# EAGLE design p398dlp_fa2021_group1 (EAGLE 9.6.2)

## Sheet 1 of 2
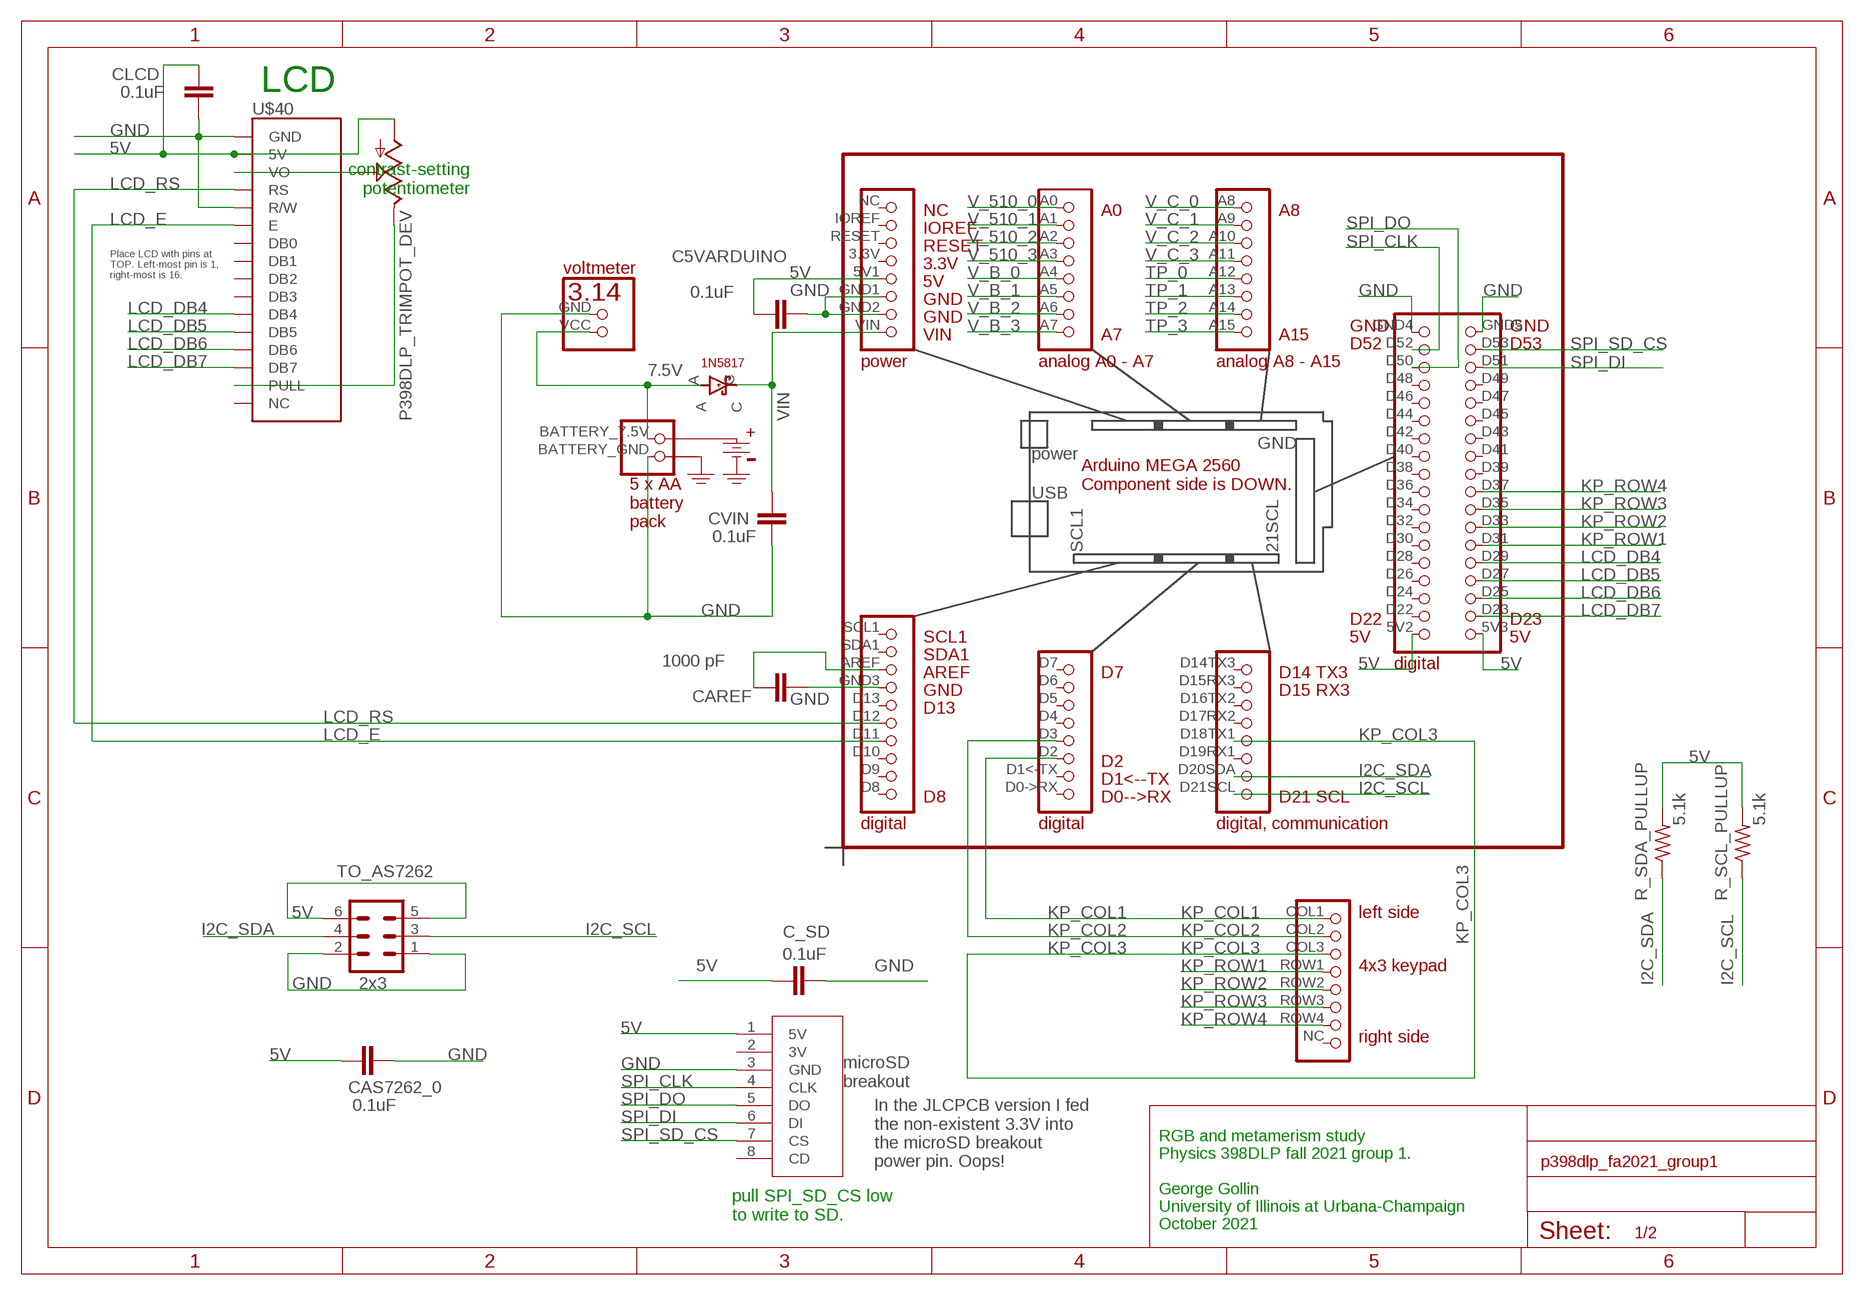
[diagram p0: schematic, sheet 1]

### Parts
C5VARDUINO  0.1uF  C5/3.5  [C5B3.5]
C_SD  0.1uF  C5/3.5  [C5B3.5]
CAREF  1000 pF  C5/3.5  [C5B3.5]
CAS7262_0  0.1uF  C5/3.5  [C5B3.5]
CLCD  0.1uF  C5/3.5  [C5B3.5]
CVIN  0.1uF  C5/3.5  [C5B3.5]
DIODE1  P398DLP_1N5817_DEV  [P398DLP_1N5817_PKG]
R_SCL_PULLUP  5.1k  R-US_0207/7  [0207/7]
R_SDA_PULLUP  5.1k  R-US_0207/7  [0207/7]
TO_AS7262  2x3  P398DLP_RIBBON_PCB_2X3_DEV  [06V]
U$1  P398DLP_5XAA_BATTERY_DEV  [P398DLP_5XAA_BATTERY_PKG]
U$2  P398DLP_KEYPAD_DEV  [P398DLP_KEYPAD_PKG]
U$3  P398DLP_VOLTMETER_DEV  [P398DLP_VOLTMETER_PKG]
U$5  P398DLP_ARDUINO_MEGA2560_DEV  [P398DLP_ARDUINO_MEGA2560_PKG]
U$19  P398DLP_TRIMPOT_DEV  [P398DLP_TRIMPOT_PKG]
U$40  P398DLP_LCD_16X2_DEV  [P398DLP_LCD_16X2_PKG]
U$MICROSD  P398DLP_MICROSD_DEV  [P398DLP_MICROSD_PKG]

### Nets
5V [power]: C5VARDUINO.1 C_SD.2 CAS7262_0.1 CLCD.1 R_SCL_PULLUP.2 R_SDA_PULLUP.2 TO_AS7262.5 TO_AS7262.6 U$5.5V1 U$5.5V2 U$5.5V3 U$19.BOTTOM U$40.5V U$MICROSD.1(5V) ; also sheet 2
7.5V [power]: DIODE1.A U$1.BATTERY_7.5V U$3.VCC
AREF: CAREF.1 U$5.AREF
GND [power]: C5VARDUINO.2 C_SD.1 CAREF.2 CAS7262_0.2 CLCD.2 CVIN.1 TO_AS7262.1 TO_AS7262.2 U$1.BATTERY_GND U$3.GND U$5.GND1 U$5.GND2 U$5.GND3 U$5.GND4 U$5.GND5 U$40.GND U$40.R/W U$MICROSD.3(GND) ; also sheet 2
I2C_SCL: R_SCL_PULLUP.1 TO_AS7262.3 U$5.D21SCL ; also sheet 2
I2C_SDA: R_SDA_PULLUP.1 TO_AS7262.4 U$5.D20SDA ; also sheet 2
KP_COL1: U$2.COL1 U$5.D2
KP_COL2: U$2.COL2 U$5.D3
KP_COL3: U$2.COL3 U$5.D18TX1
KP_ROW1: U$2.ROW1 U$5.D31
KP_ROW2: U$2.ROW2 U$5.D33
KP_ROW3: U$2.ROW3 U$5.D35
KP_ROW4: U$2.ROW4 U$5.D37
LCD_DB4: U$5.D29 U$40.DB4
LCD_DB5: U$5.D27 U$40.DB5
LCD_DB6: U$5.D25 U$40.DB6
LCD_DB7: U$5.D23 U$40.DB7
LCD_E: U$5.D11 U$40.E
LCD_RS: U$5.D12 U$40.RS
LCD_VEE: U$19.TOP U$40.PULL
N$6: U$19.TAP U$40.VO
SPI_CLK: U$5.D52 U$MICROSD.4(CLK)
SPI_DI: U$5.D51 U$MICROSD.6(DI)
SPI_DO: U$5.D50 U$MICROSD.5(DO)
SPI_SD_CS: U$5.D53 U$MICROSD.7(CS)
TP_0: U$5.A12 ; also sheet 2
TP_1: U$5.A13 ; also sheet 2
TP_2: U$5.A14 ; also sheet 2
TP_3: U$5.A15 ; also sheet 2
V_510_0: U$5.A0 ; also sheet 2
V_510_1: U$5.A1 ; also sheet 2
V_510_2: U$5.A2 ; also sheet 2
V_510_3: U$5.A3 ; also sheet 2
V_B_0: U$5.A4 ; also sheet 2
V_B_1: U$5.A5 ; also sheet 2
V_B_2: U$5.A6 ; also sheet 2
V_B_3: U$5.A7 ; also sheet 2
V_C_0: U$5.A8 ; also sheet 2
V_C_1: U$5.A9 ; also sheet 2
V_C_2: U$5.A10 ; also sheet 2
V_C_3: U$5.A11 ; also sheet 2
VIN: CVIN.2 DIODE1.C U$5.VIN
Unconnected: U$2.NC U$5.3.3V U$5.D0->RX U$5.D1<-TX U$5.D4 U$5.D5 U$5.D6 U$5.D7 U$5.D8 U$5.D9 U$5.D10 U$5.D13 U$5.D14TX3 U$5.D15RX3 U$5.D16TX2 U$5.D17RX2 U$5.D19RX1 U$5.D22 U$5.D24 U$5.D26 U$5.D28 U$5.D30 U$5.D32 U$5.D34 U$5.D36 U$5.D38 U$5.D39 U$5.D40 U$5.D41 U$5.D42 U$5.D43 U$5.D44 U$5.D45 U$5.D46 U$5.D47 U$5.D48 U$5.D49 U$5.IOREF U$5.NC U$5.RESET U$5.SCL1 U$5.SDA1 U$40.DB0 U$40.DB1 U$40.DB2 U$40.DB3 U$40.NC U$MICROSD.2(3V) U$MICROSD.8(CD)

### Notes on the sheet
- LCD
- contrast-setting
  potentiometer
- Place LCD with pins at 
  TOP. Left-most pin is 1, 
  right-most is 16.
- In the JLCPCB version I fed 
  the non-existent 3.3V into 
  the microSD breakout 
  power pin. Oops!
- pull SPI_SD_CS low
  to write to SD.
- RGB and metamerism study
  Physics 398DLP fall 2021 group 1.
  
  George Gollin
  University of Illinois at Urbana-Champaign
  October 2021

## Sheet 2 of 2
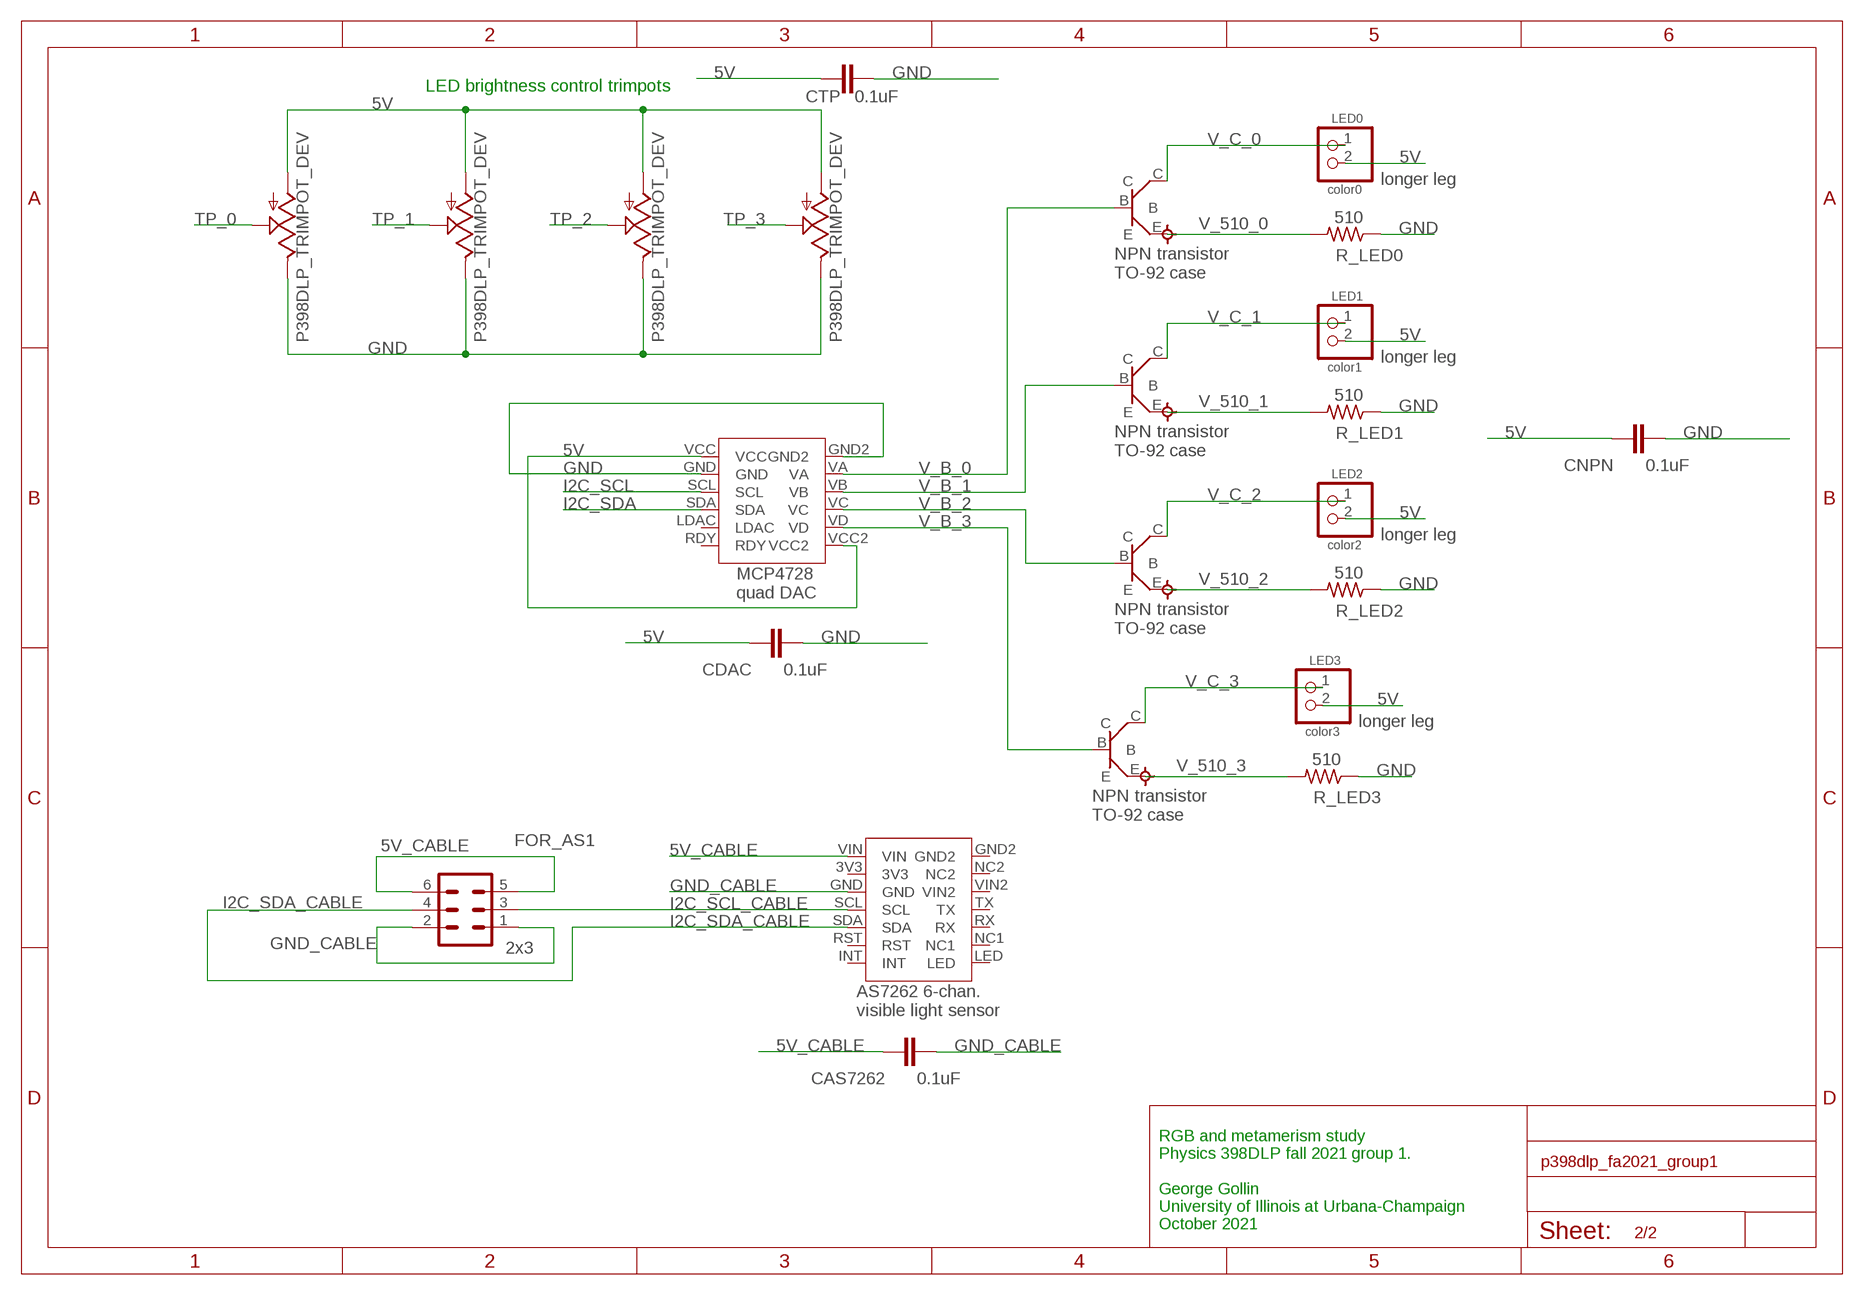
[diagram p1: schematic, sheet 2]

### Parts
CAS7262  0.1uF  C5/3.5  [C5B3.5]
CDAC  0.1uF  C5/3.5  [C5B3.5]
CNPN  0.1uF  C5/3.5  [C5B3.5]
CTP  0.1uF  C5/3.5  [C5B3.5]
FOR_AS1  2x3  P398DLP_RIBBON_PCB_2X3_DEV  [06V]
LED0  color0  PINHD-1X2  [1X02]
LED1  color1  PINHD-1X2  [1X02]
LED2  color2  PINHD-1X2  [1X02]
LED3  color3  PINHD-1X2  [1X02]
NPN0  P398DLP_NPN_DEV  [P398DLP_NPN_PKG]
NPN1  P398DLP_NPN_DEV  [P398DLP_NPN_PKG]
NPN2  P398DLP_NPN_DEV  [P398DLP_NPN_PKG]
NPN3  P398DLP_NPN_DEV  [P398DLP_NPN_PKG]
R_LED0  510  R-US_0207/7  [0207/7]
R_LED1  510  R-US_0207/7  [0207/7]
R_LED2  510  R-US_0207/7  [0207/7]
R_LED3  510  R-US_0207/7  [0207/7]
U$4  P398DLP_AS7262_DEV  [P398DLP_AS7262_PKG]
U$6  P398DLP_MCP4728_DEV  [P398DLP_MCP4728_PKG]
U$8  P398DLP_TRIMPOT_DEV  [P398DLP_TRIMPOT_PKG]
U$12  P398DLP_TRIMPOT_DEV  [P398DLP_TRIMPOT_PKG]
U$13  P398DLP_TRIMPOT_DEV  [P398DLP_TRIMPOT_PKG]
U$14  P398DLP_TRIMPOT_DEV  [P398DLP_TRIMPOT_PKG]

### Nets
5V [power]: CDAC.2 CNPN.2 CTP.2 LED0.2 LED1.2 LED2.2 LED3.2 U$6.VCC U$6.VCC2 U$8.BOTTOM U$12.BOTTOM U$13.BOTTOM U$14.BOTTOM ; also sheet 1
5V_CABLE: CAS7262.2 FOR_AS1.5 FOR_AS1.6 U$4.VIN
GND [power]: CDAC.1 CNPN.1 CTP.1 R_LED0.1 R_LED1.1 R_LED2.1 R_LED3.1 U$6.GND U$6.GND2 U$8.TOP U$12.TOP U$13.TOP U$14.TOP ; also sheet 1
GND_CABLE: CAS7262.1 FOR_AS1.1 FOR_AS1.2 U$4.GND
I2C_SCL: U$6.SCL ; also sheet 1
I2C_SCL_CABLE: FOR_AS1.3 U$4.SCL
I2C_SDA: U$6.SDA ; also sheet 1
I2C_SDA_CABLE: FOR_AS1.4 U$4.SDA
TP_0: U$8.TAP ; also sheet 1
TP_1: U$12.TAP ; also sheet 1
TP_2: U$13.TAP ; also sheet 1
TP_3: U$14.TAP ; also sheet 1
V_510_0: NPN0.E R_LED0.2 ; also sheet 1
V_510_1: NPN1.E R_LED1.2 ; also sheet 1
V_510_2: NPN2.E R_LED2.2 ; also sheet 1
V_510_3: NPN3.E R_LED3.2 ; also sheet 1
V_B_0: NPN0.B U$6.VA ; also sheet 1
V_B_1: NPN1.B U$6.VB ; also sheet 1
V_B_2: NPN2.B U$6.VC ; also sheet 1
V_B_3: NPN3.B U$6.VD ; also sheet 1
V_C_0: LED0.1 NPN0.C ; also sheet 1
V_C_1: LED1.1 NPN1.C ; also sheet 1
V_C_2: LED2.1 NPN2.C ; also sheet 1
V_C_3: LED3.1 NPN3.C ; also sheet 1
Unconnected: U$4.3V3 U$4.GND2 U$4.INT U$4.LED U$4.NC1 U$4.NC2 U$4.RST U$4.RX U$4.TX U$4.VIN2 U$6.LDAC U$6.RDY

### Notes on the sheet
- LED brightness control trimpots
- longer leg
- longer leg
- longer leg
- longer leg
- RGB and metamerism study
  Physics 398DLP fall 2021 group 1.
  
  George Gollin
  University of Illinois at Urbana-Champaign
  October 2021

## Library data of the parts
C5VARDUINO C_SD CAREF CAS7262 CAS7262_0 CDAC CLCD CNPN CTP CVIN = capacitor-wima:C: CAPACITOR
DIODE1 = p398dlp:P398DLP_1N5817_DEV: 1N5817 Schottky barrier diode
FOR_AS1 TO_AS7262 = p398dlp:P398DLP_RIBBON_PCB_2X3_DEV: CONNECTOR; OC_FARNELL: unknown; OC_NEWARK: unknown
LED0 LED1-LED3 = p398dlp_sp2020:PINHD-1X2: PIN HEADER
NPN0 NPN1-NPN3 = p398dlp:P398DLP_NPN_DEV: NPN transistor, TO-92 case
R_LED0 R_LED1-R_LED3 R_SCL_PULLUP R_SDA_PULLUP = resistor:R-US_: RESISTOR, American symbol
U$1 = p398dlp:P398DLP_5XAA_BATTERY_DEV: 5 x AA battery case
U$2 = p398dlp:P398DLP_KEYPAD_DEV: 3x4 telephone-style keypad
U$3 = p398dlp:P398DLP_VOLTMETER_DEV: Adafruit 2-wire voltmeter
U$4 = p398dlp:P398DLP_AS7262_DEV: AS7262 6 channel visible light sensor
U$5 = p398dlp:P398DLP_ARDUINO_MEGA2560_DEV: Arduino MEGA 2560, component side DOWN
U$6 = p398dlp:P398DLP_MCP4728_DEV: MCP4725 12-bit DACMCP4728 quad 12-bit DAC Adafriuit 4470
U$8 U$12-U$14 U$19 = p398dlp_fa2020:P398DLP_TRIMPOT_DEV: trimpot
U$40 = p398dlp:P398DLP_LCD_16X2_DEV: 2x16 liquid crystal display, four mounting holes
U$MICROSD = p398dlp_sp2020:P398DLP_MICROSD_DEV: Adafruit microSD reader breakout board

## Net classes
1 power: width 0.305 mm

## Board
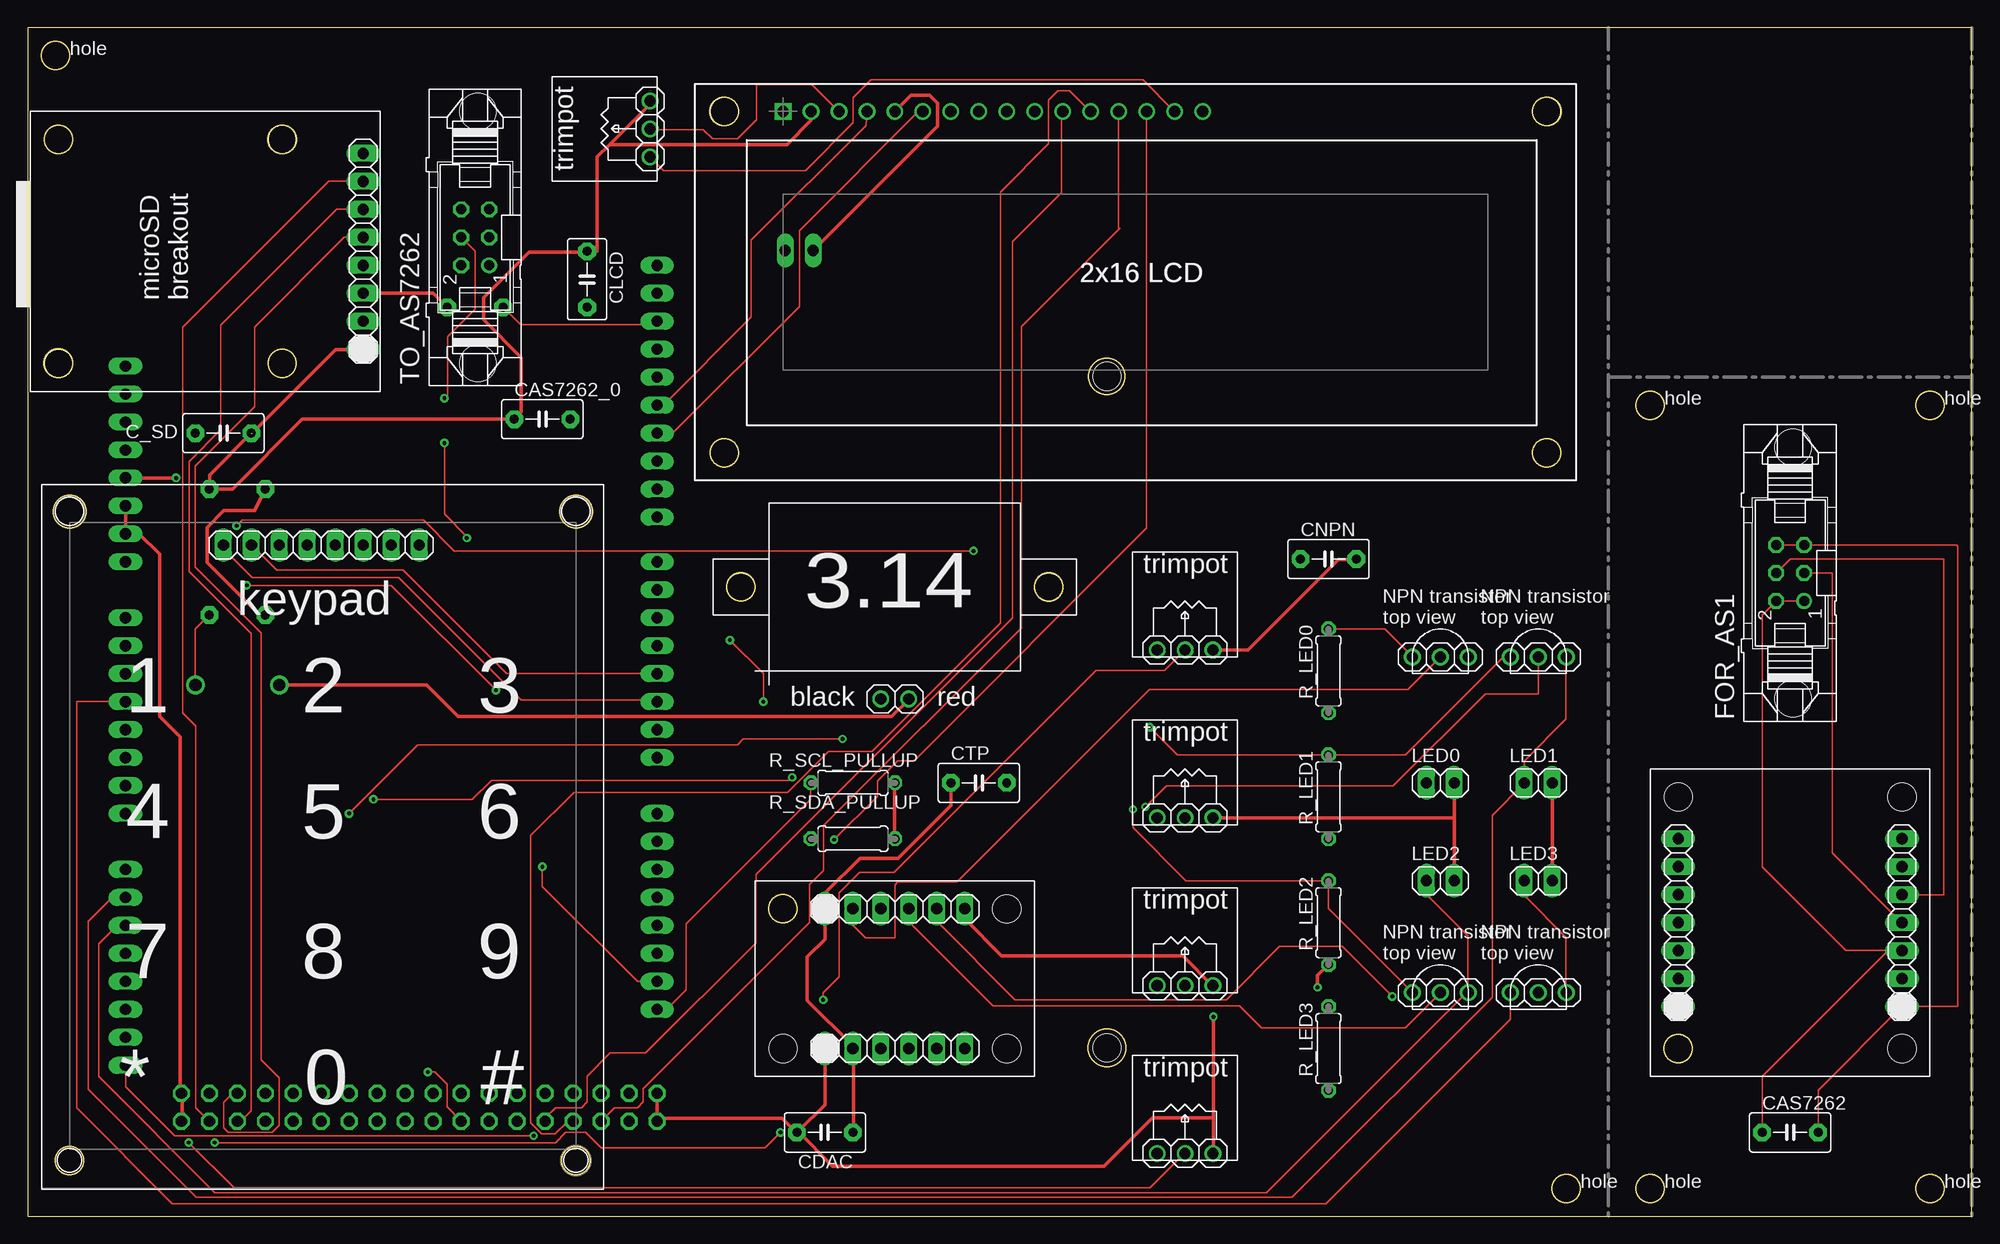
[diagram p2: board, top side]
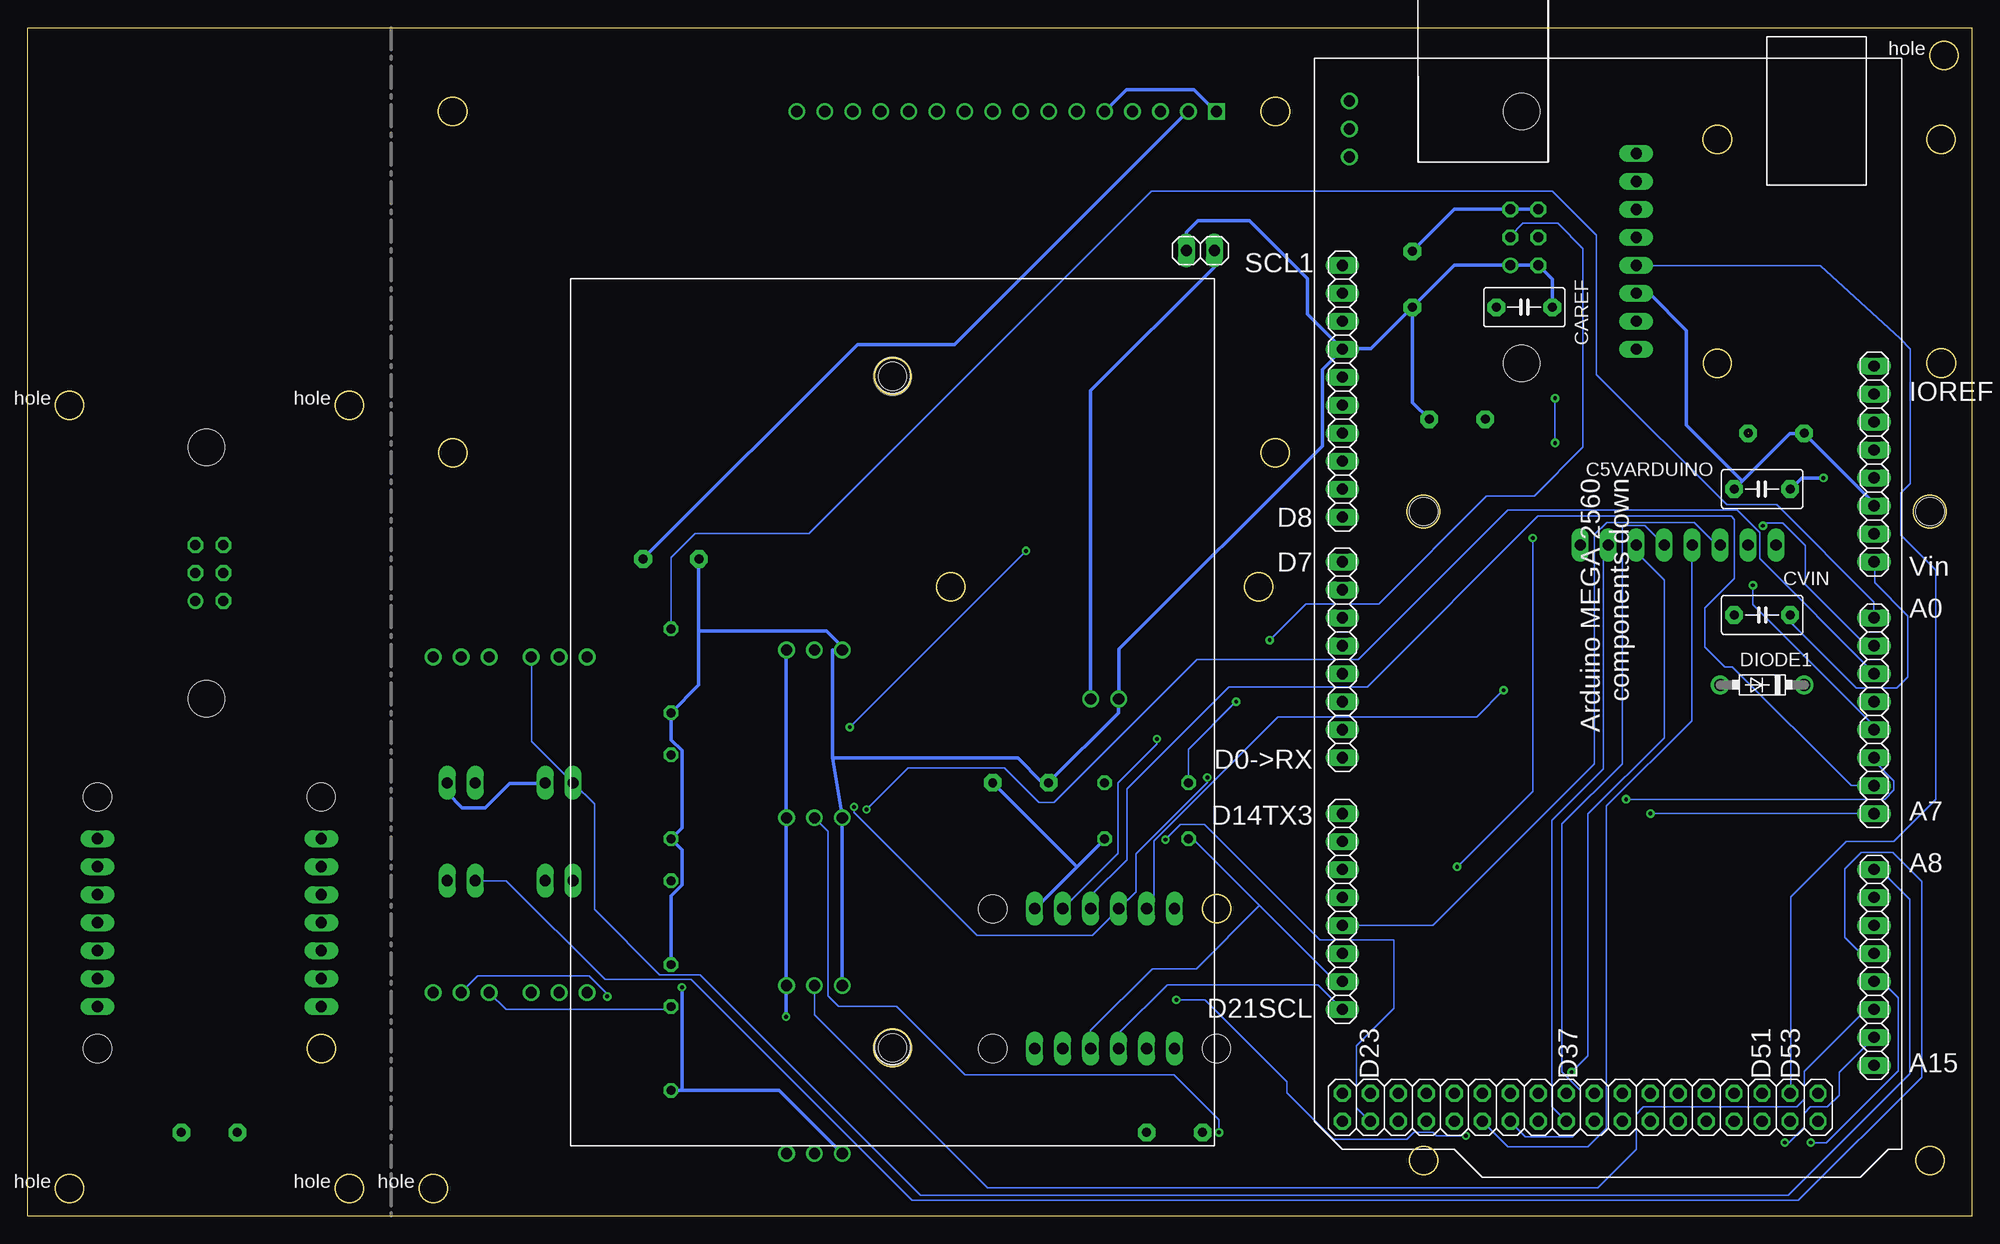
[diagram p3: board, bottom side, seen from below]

Size 176.53 x 107.95 mm. Coordinates in mm from the lower left corner, seen from the top.
Outline: 0,0 176.53,0 176.53,107.95 0,107.95 0,0
Copper layers (1*16): Top 0.035mm / dielectric 1.5mm / Bottom 0.035mm
Design rules "default": minimum track width 6mil, minimum drill 0.35mm, track to track 6mil, track to pad 6mil, pad to pad 6mil, via to via 6mil, smd to smd 6mil, copper to edge 40mil, drill to drill 6mil, minimum pad ring 10mil, minimum via ring 8mil, stop-mask expansion 4mil, vias tented up to drill 0mil, thermal gap 10mil

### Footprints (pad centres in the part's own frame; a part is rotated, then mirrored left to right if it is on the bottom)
C5B3.5 = drill 0.813 pad 1.6 octagon: 1 -2.54,0; 2 2.54,0
P398DLP_1N5817_PKG = drill 1.1 pad 1.7: A -3.81,0; C 3.81,0
06V = drill 0.914: 1 -2.54,-1.27 | drill 0.914 octagon: 2 -2.54,1.27; 3 0,-1.27; 4 0,1.27; 5 2.54,-1.27; 6 2.54,1.27 | hole 3.302: 11.43,-0.254; -11.43,-0.254
1X02 = drill 1.016 long: 1 -1.27,0; 2 1.27,0
P398DLP_NPN_PKG = drill 1.016: B 0,0; C 2.54,0; E -2.54,0
0207/7 = drill 0.813 octagon: 1 -3.81,0; 2 3.81,0
P398DLP_5XAA_BATTERY_PKG = drill 1.016 long: BATTERY_7.5V 0,-2.54; BATTERY_GND 2.54,-2.54 | hole 2.54: 29.21,69.85; 29.21,8.89
P398DLP_KEYPAD_PKG = drill 1.016 long: COL1 0,0; COL2 2.54,0; COL3 5.08,0; NC 17.78,0; ROW1 7.62,0; ROW2 10.16,0; ROW3 12.7,0; ROW4 15.24,0 | hole 2.54: -13.97,3.048; 32.004,3.048; 32.004,-55.88; -13.97,-55.88
P398DLP_VOLTMETER_PKG = drill 1.016: GND 10.16,-2.54; VCC 12.7,-2.54 | hole 2.54: -2.54,7.62; 25.4,7.62
P398DLP_AS7262_PKG = drill 1.016 long: 3V3 8.89,2.54; GND 11.43,2.54; GND2 6.35,22.86; INT 21.59,2.54; LED 21.59,22.86; NC1 19.05,22.86; NC2 8.89,22.86; RST 19.05,2.54; RX 16.51,22.86; SCL 13.97,2.54; SDA 16.51,2.54; TX 13.97,22.86; VIN 6.35,2.54; VIN2 11.43,22.86 | hole 2.54: 2.54,22.86; 25.4,2.54; 25.4,22.86; 2.54,2.54
P398DLP_ARDUINO_MEGA2560_PKG = drill 1.016 long: 3.3V 35.56,50.8; 5V1 38.1,50.8; A0 50.8,50.8; A1 53.34,50.8; A2 55.88,50.8; A3 58.42,50.8; A4 60.96,50.8; A5 63.5,50.8; A6 66.04,50.8; A7 68.58,50.8; A8 73.66,50.8; A9 76.2,50.8; A10 78.74,50.8; A11 81.28,50.8; A12 83.82,50.8; A13 86.36,50.8; A14 88.9,50.8; A15 91.44,50.8; AREF 23.876,2.54; D0->RX 63.5,2.54; D1<-TX 60.96,2.54; D2 58.42,2.54; D3 55.88,2.54; D4 53.34,2.54; D5 50.8,2.54; D6 48.26,2.54; D7 45.72,2.54; D8 41.656,2.54; D9 39.116,2.54; D10 36.576,2.54; D11 34.036,2.54; D12 31.496,2.54; D13 28.956,2.54; D14TX3 68.58,2.54; D15RX3 71.12,2.54; D16TX2 73.66,2.54; D17RX2 76.2,2.54; D18TX1 78.74,2.54; D19RX1 81.28,2.54; D20SDA 83.82,2.54; D21SCL 86.36,2.54; GND1 40.64,50.8; GND2 43.18,50.8; GND3 26.416,2.54; IOREF 30.48,50.8; NC 27.94,50.8; RESET 33.02,50.8; SCL1 18.796,2.54; SDA1 21.336,2.54; VIN 45.72,50.8 | drill 1.016 octagon: 5V2 93.98,2.54; 5V3 96.52,2.54; D22 93.98,5.08; D23 96.52,5.08; D24 93.98,7.62; D25 96.52,7.62; D26 93.98,10.16; D27 96.52,10.16; D28 93.98,12.7; D29 96.52,12.7; D30 93.98,15.24; D31 96.52,15.24; D32 93.98,17.78; D33 96.52,17.78; D34 93.98,20.32; D35 96.52,20.32; D36 93.98,22.86; D37 96.52,22.86; D38 93.98,25.4; D39 96.52,25.4; D40 93.98,27.94; D41 96.52,27.94; D42 93.98,30.48; D43 96.52,30.48; D44 93.98,33.02; D45 96.52,33.02; D46 93.98,35.56; D47 96.52,35.56; D48 93.98,38.1; D49 96.52,38.1; D50 93.98,40.64; D51 96.52,40.64; D52 93.98,43.18; D53 96.52,43.18; GND4 93.98,45.72; GND5 96.52,45.72
P398DLP_MCP4728_PKG = drill 1.016 long: GND 8.89,2.54; GND2 6.35,15.24; LDAC 16.51,2.54; RDY 19.05,2.54; SCL 11.43,2.54; SDA 13.97,2.54; VA 8.89,15.24; VB 11.43,15.24; VC 13.97,15.24; VCC 6.35,2.54; VCC2 19.05,15.24; VD 16.51,15.24 | hole 2.54: 2.54,15.24; 22.86,2.54; 22.86,15.24; 2.54,2.54
P398DLP_MOUNTING_HOLE_PKG = hole 2.54: 0,0
P398DLP_TRIMPOT_PKG = drill 1.016: BOTTOM 7.303,0.635; TAP 4.763,0.635; TOP 2.223,0.635
P398DLP_LCD_16X2_PKG = drill 1.016: 5V 2.544,0.006; DB0 15.244,0.006; DB1 17.784,0.006; DB2 20.324,0.006; DB3 22.864,0.006; DB4 25.404,0.006; DB5 27.944,0.006; DB6 30.484,0.006; DB7 33.024,0.006; E 12.704,0.006; NC 38.104,0.006; PULL 35.564,0.006; R/W 10.164,0.006; RS 7.624,0.006; VO 5.084,0.006 | drill 1.016 square: GND 0.004,0.006 | hole 2.54: -5.334,0; -5.334,-30.988; 69.342,-30.988; 69.342,0
P398DLP_MICROSD_PKG = drill 1.016 long: 1 0,0; 2 2.54,0; 3 5.08,0; 4 7.62,0; 5 10.16,0; 6 12.7,0; 7 15.24,0; 8 17.78,0 | hole 2.54: -1.27,27.686; 19.05,27.686; 19.05,7.366; -1.27,7.366

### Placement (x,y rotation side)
C5VARDUINO  19.05,66.04 180 bottom
C_SD  17.78,71.12 0 top
CAREF  40.64,82.55 0 bottom
CAS7262  160.02,7.62 0 top
CAS7262_0  46.74,72.39 0 top
CDAC  72.39,7.62 180 top
CLCD  50.8,85.09 270 top
CNPN  118.11,59.69 0 top
CTP  86.36,39.37 0 top
CVIN  19.05,54.61 0 bottom
DIODE1  19.05,48.26 0 bottom
FOR_AS1  160.02,58.42 90 top
LED0  128.27,39.37 0 top
LED1  137.16,39.37 0 top
LED2  128.27,30.48 0 top
LED3  137.16,30.48 0 top
NPN0  128.27,50.8 0 top
NPN1  137.16,50.8 0 top
NPN2  128.27,20.32 0 top
NPN3  137.16,20.32 0 top
R_LED0  118.11,49.53 90 top
R_LED1  118.11,38.1 90 top
R_LED2  118.11,26.67 90 top
R_LED3  118.11,15.24 90 top
R_SCL_PULLUP  74.93,39.37 0 top
R_SDA_PULLUP  74.93,34.29 0 top
TO_AS7262  40.64,88.9 90 top
U$1  68.78,85.17 180 bottom
U$2  17.78,60.96 0 top
U$3  67.31,49.53 0 top
U$4  172.72,12.7 90 top
U$5  59.69,105.16 270 bottom
U$6  66.04,12.7 0 top
U$7  [P398DLP_MOUNTING_HOLE_PKG]  172.72,2.54 0 top
U$8  100.33,5.08 0 top
U$9  [P398DLP_MOUNTING_HOLE_PKG]  172.72,73.66 0 top
U$10  [P398DLP_MOUNTING_HOLE_PKG]  147.32,73.66 0 top
U$11  [P398DLP_MOUNTING_HOLE_PKG]  147.32,2.54 0 top
U$12  100.33,20.32 0 top
U$13  100.33,35.56 0 top
U$14  100.33,50.8 0 top
U$19  57.15,93.98 90 top
U$40  68.58,100.33 0 top
U$60  [P398DLP_MOUNTING_HOLE_PKG]  2.54,105.41 0 top
U$64  [P398DLP_MOUNTING_HOLE_PKG]  139.7,2.54 0 top
U$MICROSD  30.48,78.74 90 top

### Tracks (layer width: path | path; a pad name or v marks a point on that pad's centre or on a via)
5V  (via drill 0.35)  (1 unrouted)
  Top 0.305: v13.49,67.06 U$5.5V1 | 52.83,97.33 51.71,96.22 51.71,87.63 CLCD.1 50.67,87.55 45.52,87.55 41.4,83.44 41.4,81.41 44.83,77.98 44.83,73.03 CAS7262_0.1 24.94,72.39 18.62,66.06 16.54,66.06 | 52.83,97.33 56.46,100.97 56.46,101.27 U$19.BOTTOM | U$40.5V 71.12,99.52 68.94,97.33 52.83,97.33 | 16.54,66.06 C5VARDUINO.1 | LED0.2 129.54,36.2 | 129.54,36.2 LED2.2 | LED3.2 138.46,30.48 138.46,39.32 LED1.2 | U$5.5V2 U$5.5V3 57.43,8.91 68.5,8.91 69.72,7.7 CDAC.2 69.88,7.62 69.96,7.71 | U$6.VCC 72.39,10.13 69.96,7.71 | R_SDA_PULLUP.2 78.72,34.29 78.72,39.32 R_SCL_PULLUP.2 | v107.67,18.14 107.67,8.94 | 107.67,8.94 107.67,5.71 U$8.BOTTOM | U$14.BOTTOM 110.8,51.44 119.02,59.66 120.62,59.66 CNPN.2 | U$6.VCC2 85.09,27.03 88.44,23.67 104.88,23.67 107.59,20.95 U$12.BOTTOM | 69.96,7.71 73.1,4.57 97.74,4.57 102.11,8.94 107.67,8.94 | U$13.BOTTOM 129.54,36.2 | 20.34,71.09 27.96,78.72 30.48,78.72 U$MICROSD.1 | C_SD.2 16.54,67.33 16.54,66.06
  Bottom 0.305: v13.49,67.06 15.47,67.06 16.46,66.06 C5VARDUINO.1 | LED1.2 138.43,38.48 137.06,37.11 134.98,37.11 132.77,39.32 129.54,39.32 LED0.2 | 81.27,31.74 78.72,34.29 R_SDA_PULLUP.2 | 81.27,31.74 85.04,27.96 U$6.VCC2 | 81.27,31.74 CTP.2 | TO_AS7262.6 TO_AS7262.5 46.99,91.44 CLCD.1 | v107.67,18.14 107.67,20.95 U$12.BOTTOM 107.67,21.03 107.67,36.2 U$13.BOTTOM 107.67,36.27 107.67,51.44 U$14.BOTTOM | U$40.5V 71.17,100.28 71.27,100.28 92.38,79.17 101.19,79.17 120.62,59.74 CNPN.2
5V_CABLE
  Top 0.152: CAS7262.2 162.56,11.43 U$4.VIN 175.26,19.05 175.26,60.83 175.13,60.96 FOR_AS1.5 FOR_AS1.6
7.5V
  Top 0.305: DIODE1.A 22.86,48.23 36.25,48.23 39.09,45.39 78.46,45.39 80.01,46.94 U$3.VCC
  Bottom 0.305: U$3.VCC 80.01,74.98 68.78,86.21 U$1.BATTERY_7.5V
AREF
  Top 0.152: U$5.AREF 57.4,81.03 57.4,80.97 44.76,80.97 CAREF.1
GND  (via drill 0.35)
  Top 0.305: CDAC.1 74.98,7.62 74.98,15.24 U$6.GND 74.93,15.47 70.79,19.61 70.79,23.55 72.39,25.15 U$6.GND2 72.47,28.04 72.47,29.41 75.56,32.51 79.02,32.51 83.82,37.31 CTP.1 | v117.12,20.8 117.12,21.87 R_LED2.1 | U$1.BATTERY_GND 82.63,99.01 82.63,101.07 81.89,101.8 80.21,101.8 U$40.R/W | U$MICROSD.3 36.83,83.82 CAREF.2 | U$5.GND5 14.02,8.69 14.02,11.12 U$5.GND4 13.87,11.28 13.87,43.54 12.01,45.39 12.01,60.12 10.16,61.98 U$5.GND2 8.91,62.03 8.91,64.47 U$5.GND1 | CVIN.1 21.08,54.61 16.31,59.38 16.31,62.56 17.83,64.08 20.61,64.08 C5VARDUINO.2
  Bottom 0.305: 117.12,11.43 108.28,11.43 102.56,5.71 U$8.TOP | 117.12,11.43 R_LED3.1 | U$12.TOP 102.56,20.95 102.56,36.2 U$13.TOP 103.45,41.6 | 103.45,41.6 103.45,51.44 U$14.TOP 102.55,51.7 103.99,53.14 115.59,53.14 | R_LED2.1 118.11,29.11 117.12,30.1 117.12,33.3 R_LED1.1 117.12,35.28 117.12,42.29 118.11,43.28 R_LED0.1 115.59,48.23 115.59,53.14 | 115.59,53.14 115.59,59.66 CNPN.1 | 103.45,41.6 86.59,41.6 84.45,39.47 83.9,39.47 CTP.1 83.82,39.4 77.5,45.72 77.5,46.94 U$3.GND 77.42,47.09 77.42,51.51 58.98,69.95 58.98,76.89 57.23,78.64 U$5.GND3 | v117.12,20.8 117.12,11.43 | U$40.GND 68.66,100.36 68.68,100.36 70.64,102.31 76.76,102.31 78.72,100.36 U$40.R/W | CLCD.2 54.56,78.79 57.15,78.79 U$5.GND3 | U$1.BATTERY_GND 71.32,89.38 70.28,90.42 65.61,90.42 60.33,85.14 60.33,81.92 U$5.GND3 | C5VARDUINO.2 20.85,66.78 | 20.85,66.78 16.54,71.09 15.24,71.09 C_SD.1 15.16,71.02 8.91,64.77 8.91,64.54 U$5.GND1 | U$MICROSD.3 29.31,83.82 25.93,80.44 25.93,71.86 20.85,66.78 | CAREF.2 38.1,85.09 TO_AS7262.2 TO_AS7262.1 46.99,86.36 CLCD.2 | CLCD.2 50.8,73.91 CAS7262_0.2
GND_CABLE
  Top 0.152: 168.91,24.16 170.16,24.16 U$4.GND | CAS7262.1 157.48,12.72 168.91,24.16 | FOR_AS1.1 FOR_AS1.2 157.48,54.61 157.48,31.75 165.07,24.16 168.91,24.16
I2C_SCL  (via drill 0.35)
  Top 0.152: U$5.D21SCL 58.01,18.8 59.79,20.57 59.79,26.57 71.09,37.87 71.09,39.32 R_SCL_PULLUP.1 | v63.75,52.32 66.8,49.28 v66.8,46.74
  Bottom 0.152: U$6.SCL 77.42,15.24 77.42,16.66 73.05,21.03 59.36,21.03 57.15,18.82 U$5.D21SCL | TO_AS7262.3 41.91,89.03 40.77,90.17 37.59,90.17 35.31,87.88 35.31,69.85 39.75,65.41 44.07,65.41 53.85,55.63 60.45,55.63 v63.75,52.32 | v66.8,46.74 71.12,42.42 R_SCL_PULLUP.1
I2C_SCL_CABLE
  Top 0.152: U$4.SCL 163.83,33.02 163.83,58.42 FOR_AS1.3
I2C_SDA  (via drill 0.35)
  Top 0.152: U$5.D20SDA 55.37,21.34 46.74,29.97 v46.74,31.75 | TO_AS7262.4 40.64,87.63 40.64,82.36 38.15,79.88 38.15,74.6 v37.85,74.3 | v39.88,61.59 39.88,61.72 37.85,63.75 v37.85,70.23
  Bottom 0.152: R_SDA_PULLUP.1 70.74,34.29 64.61,28.16 | U$5.D20SDA 57.78,21.34 64.67,28.22 70.41,22.48 74.42,22.48 80.01,16.89 U$6.SDA | v46.74,31.75 39.88,38.61 v39.88,61.59 | v37.85,74.3 v37.85,70.23
I2C_SDA_CABLE
  Top 0.152: U$4.SDA 173.99,29.21 173.99,59.69 160.02,59.69 FOR_AS1.4
KP_COL1
  Top 0.152: U$2.COL1 17.78,60.63 20.4,58.01 33.71,58.01 44.81,46.91 57.15,46.91 U$5.D2
KP_COL2
  Top 0.152: U$5.D3 57.15,49.3 43.51,49.3 34.11,58.7 22.61,58.7 20.34,60.96 U$2.COL2
KP_COL3
  Bottom 0.152: U$2.COL3 23.16,60.96 25.22,63.02 33.15,63.02 34.27,61.9 34.27,41.07 48.92,26.42 U$5.D18TX1
KP_ROW1
  Bottom 0.152: U$5.D31 42.11,6.3 34.87,6.3 33.17,8 33.17,37.26 25.45,44.98 25.45,60.96 U$2.ROW1
KP_ROW2
  Bottom 0.152: 28.27,60.96 U$2.ROW2 29.69,62.71 31.75,62.71 31.75,41.1 37.21,35.64 37.21,13.11 35.56,11.46 35.56,7.98 36.3,7.24 40.54,7.24 41.91,8.61 U$5.D33
KP_ROW3  (via drill 0.35)
  Top 0.152: v36.35,13.11 36.98,13.11 38.08,12.01 38.08,9.93 U$5.D35
  Bottom 0.152: U$2.ROW3 30.48,60.33 27.94,57.78 27.94,43.46 34.87,36.52 34.87,14.58 v36.35,13.11
KP_ROW4
  Bottom 0.152: U$5.D37 38.12,9.93 38.12,35.94 33.45,40.62 33.45,60.96 U$2.ROW4
LCD_DB4
  Top 0.152: U$5.D29 46.99,8.94 47.93,9.88 50.29,9.88 50.8,10.39 50.8,12.72 52.91,14.83 56.13,14.83 66.14,24.84 66.14,31.06 89.41,54.33 89.41,88.49 93.88,92.97 93.88,100.24 U$40.DB4
LCD_DB5
  Top 0.152: U$5.D27 49.53,8.61 49.02,8.61 47.9,7.49 46.69,7.49 45.7,8.48 45.7,34.59 49.61,38.51 68.99,38.51 72.72,42.24 76.68,42.24 88.34,53.9 88.34,93.02 92.71,97.38 92.71,101.37 93.57,102.23 94.59,102.23 96.47,100.36 U$40.DB5
LCD_DB6
  Top 0.152: U$5.D25 53.31,9.88 55.4,9.88 55.91,10.39 55.91,11.58 71.02,26.7 71.02,30.12 72.29,31.39 72.29,35.48 90.22,53.42 90.22,80.77 99.18,89.74 99.06,89.74 U$40.DB6
LCD_DB7  (via drill 0.35)
  Top 0.152: v73.23,34.21 77.17,38.15 77.17,39.55 78.99,41.38 80.47,41.38 101.58,62.48 101.58,100.28 U$40.DB7
  Bottom 0.152: U$5.D23 54.66,8.64 55.88,9.86 55.88,15.47 52.48,18.87 52.48,25.12 59.21,25.12 69.67,35.59 71.86,35.59 v73.23,34.21
LCD_E
  Top 0.152: U$5.D11 58.57,71.12 70.08,82.63 70.08,89.51 80.91,100.34 U$40.E
LCD_RS
  Top 0.152: U$5.D12 57.73,73.66 65.71,81.64 65.71,88.65 76.11,99.05 U$40.RS
LCD_VEE
  Top 0.152: U$19.TOP 57.75,94.97 70.64,94.97 74.95,99.29 74.95,101.58 76.58,103.2 101.24,103.2 104.09,100.36 U$40.PULL
N$6
  Top 0.152: U$19.TAP 56.54,98.68 61.34,98.68 62.18,97.84 64.44,97.84 66.19,99.59 66.19,102.74 71.22,102.74 73.61,100.36 U$40.VO
SPI_CLK
  Bottom 0.152: U$5.D52 16.46,11.2 16.46,29.01 11.43,34.04 7.11,34.04 3.3,37.85 3.3,58.67 6.48,61.85 6.48,65.66 5.59,66.55 5.59,78.77 6.53,79.71 13.79,86.33 30.48,86.33 U$MICROSD.4
SPI_DI
  Top 0.152: U$5.D51 19.33,8.64 20.3,9.6 20.3,52.93 14.66,58.57 14.66,68.56 17.55,71.45 17.55,80.92 28.07,91.44 U$MICROSD.6
SPI_DO
  Top 0.152: U$5.D50 18.62,11.18 17.8,10.36 17.8,8.03 18.21,7.62 22.23,7.62 22.86,8.25 22.86,12.57 21.22,14.21 21.22,52.97 15.21,58.98 15.21,68.15 20.61,73.55 20.61,80.76 28.75,88.9 U$MICROSD.5
SPI_SD_CS
  Top 0.152: U$5.D53 15.27,9.88 15.27,44.53 14.1,45.7 14.1,80.75 27.33,93.98 U$MICROSD.7
TP_0  (via drill 0.35)
  Top 0.152: U$8.TAP 105.03,5.71 101.91,2.59 18.75,2.59 v14.63,6.71
  Bottom 0.152: v14.63,6.71 13.21,6.71 6.71,13.21 6.71,19.84 8.2,21.34 U$5.A12
TP_1
  Bottom 0.152: U$5.A13 9.58,18.8 15.21,13.16 15.21,10.62 15.9,9.93 29.82,9.93 30.48,9.27 30.48,6.1 33.98,2.59 89.38,2.59 105.08,18.29 U$12.TAP
TP_2  (via drill 0.35)
  Top 0.152: v16.99,6.71 47.93,6.71 48.84,7.62 50.67,7.62 52.07,6.22 66.95,6.22 v68.35,7.62
  Bottom 0.152: U$5.A14 12.06,13.08 12.06,11 13.13,9.93 14.66,9.93 15.21,9.37 15.21,8.1 16.61,6.71 v16.99,6.71 | v68.35,7.62 68.35,8.76 72.47,12.88 91.44,12.88 97.64,19.07 102.89,19.07 103.83,20.02 103.83,34.95 U$13.TAP
TP_3  (via drill 0.35)
  Top 0.152: v45.95,7.32 13.36,7.32 8.91,11.76 8.91,13.72 U$5.A15 | v72.24,19.66 72.24,20.32 73.66,21.74 73.66,29.36 75.54,31.24 78.69,31.24 97,49.55 103.2,49.55 U$14.TAP
  Bottom 0.152: v45.95,7.32 48.64,7.32 48.95,7.62 50.67,7.62 51.31,6.99 57.99,6.99 62.2,11.2 62.2,12.22 69.65,19.66 v72.24,19.66
V_510_0
  Top 0.152: R_LED0.2 123.22,53.34 125.73,50.83 NPN0.E
  Bottom 0.152: R_LED0.2 118.11,59.82 115.93,62 105.56,62 74.47,93.09 38.1,93.09 34.11,89.1 34.11,76.45 22.28,64.62 17.73,64.62 8.91,55.8 8.91,54.41 U$5.A0
V_510_1  (via drill 0.35)
  Top 0.152: NPN1.E 133.99,50.8 125.09,41.91 R_LED1.2 118.08,41.88 104.42,41.88 v101.88,44.42 | v18.97,62.71 19.48,63.22 35.94,63.22 38.73,60.43 v85.88,60.43
  Bottom 0.152: U$5.A1 9.55,51.82 15.11,57.38 15.11,60.91 17.17,62.97 18.72,62.97 v18.97,62.71 | v101.88,44.42 v85.88,60.43
V_510_2  (via drill 0.35)
  Top 0.152: NPN2.E 125.73,20.34 118.11,27.96 R_LED2.2 105.18,30.48 100.36,35.31 v100.36,36.96
  Bottom 0.152: v100.36,36.96 96.6,40.72 87.83,40.72 84.68,37.57 83.36,37.57 70.38,50.55 55.7,50.55 42.11,64.14 21.31,64.14 19.28,62.1 19.28,59.72 8.91,49.35 8.91,49.3 U$5.A2
V_510_3
  Top 0.152: U$5.A3 4.45,46.74 4.45,9.86 13.13,1.17 117.88,1.17 134.62,17.91 NPN3.E
  Bottom 0.152: R_LED3.2 118.36,18.8 133.1,18.8 NPN3.E
V_B_0  (via drill 0.35)
  Top 0.152: v19.89,57.3 32.99,57.3 v42.52,47.78 | NPN0.B 128.25,50.75 125.32,47.83 101.86,47.83 84.39,30.35 78.99,30.35 78.74,30.1 78.74,25.27 76.07,25.27 74.93,26.42 U$6.VA
  Bottom 0.152: v19.89,57.3 19.89,55.55 8.91,44.58 8.91,44.2 U$5.A4 | v42.52,47.78 44.93,45.36 62.99,45.36 74.27,34.09 74.27,28.6 U$6.VA
V_B_1  (via drill 0.35)
  Top 0.152: v31.39,37.87 40.39,37.87 42.11,39.6 69.16,39.6 v69.42,39.85 | v101.5,37.19 103.4,39.09 123.98,39.09 132.33,47.45 137.16,47.45 NPN1.B
  Bottom 0.152: v31.39,37.87 7.92,37.87 7.09,38.71 7.09,39.55 8.84,41.3 8.84,41.6 U$5.A5 | v69.42,39.85 69.42,39.4 75.92,32.89 75.92,29.46 77.42,27.96 U$6.VB 77.5,27.89 79.86,25.53 90.35,25.53 101.5,36.68 v101.5,37.19
V_B_2
  Top 0.152: U$6.VC 80.01,26.75 87.63,19.13 110.01,19.13 112.01,17.12 125.09,17.12 128.25,20.27 NPN2.B
  Bottom 0.152: U$5.A6 10.97,39.12 21.74,49.89 22.45,49.89 24.26,51.69 24.26,55.24 21.59,57.91 21.59,63.3 21.87,63.58 39.4,63.58 54.89,48.08 67.46,48.08 76.73,38.81 76.73,32.38 80.01,29.11 U$6.VC
V_B_3  (via drill 0.35)
  Top 0.152: U$6.VD 82.55,26.8 89.66,19.68 108.84,19.68 113.67,24.51 119.36,24.51 v123.9,19.96 | v29.18,36.58 35.43,42.82 64.44,42.82 64.97,43.36 v73.99,43.36
  Bottom 0.152: v123.9,19.96 123.9,20.22 125.53,21.84 135.66,21.84 137.16,20.34 NPN3.B | v29.18,36.58 U$5.A7 | v73.99,43.36 73.99,42.9 77.55,39.34 77.55,32.94 U$6.VD
V_C_0
  Bottom 0.152: U$5.A8 8.36,31.5 5.64,28.78 5.64,12.93 16.66,1.91 95.45,1.91 115.49,21.95 119.13,21.95 125.07,27.89 125.07,37.44 LED0.1 130.76,43.13 130.76,50.75 NPN0.C
V_C_1
  Top 0.152: U$5.A9 7.7,28.96 5.51,26.77 5.51,11.53 15.32,1.73 114.81,1.73 132.97,19.89 132.97,36.42 135.87,39.32 LED1.1 135.89,41.38 139.68,45.16 139.68,50.75 NPN1.C
V_C_2
  Top 0.152: LED2.1 127,29.23 130.76,25.48 130.76,20.34 NPN2.C 130.68,20.34 112.5,2.16 16.99,2.16 6.45,12.7 6.45,24.74 8.13,26.42 U$5.A10
V_C_3
  Top 0.152: LED3.1 135.89,29.13 139.68,25.35 139.68,20.34 NPN3.C
  Bottom 0.152: U$5.A11 10.08,23.88 11.56,25.35 11.56,31.55 10.06,33.05 7.19,33.05 4.57,30.43 4.57,12.65 15.75,1.47 96.24,1.47 116.28,21.51 124.1,21.51 133.07,30.48 LED3.1
VIN
  Top 0.152: DIODE1.C 15.24,53.34 CVIN.2
  Bottom 0.152: CVIN.2 16.51,53.98 10.52,47.98 6.81,47.98 5.82,48.97 5.82,54.53 8.84,57.56 8.84,59.44 U$5.VIN

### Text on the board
tDocu: battery / 7.5V | battery / GND | JLCJLCJLCJLC | pp398dlp_fa2021_group1 | long leg | long leg | long leg | long leg | pp398dlp_fa2021_group1 | Physics 398DLP group 1 / Fall 2021 / / George Gollin / University of Illinois / October 2021 / Fille de Lear Designs
bDocu: p398dlp_fa2021_group1 | battery / 7.5V | battery / GND | Physics 398DLP group 1 / Fall 2021 / George Gollin / University of Illinois / October 2021 / Fille de Lear Designs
